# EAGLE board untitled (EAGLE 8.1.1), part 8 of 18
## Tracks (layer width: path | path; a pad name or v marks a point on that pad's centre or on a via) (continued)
S$7704 (continued)
  Bottom 0: 276.47,99.72 276.52,99.67
S$7705
  Bottom 0: 276.52,99.67 276.59,99.63
S$7706
  Bottom 0: 276.59,99.63 276.65,99.61
S$7707
  Bottom 0: 276.65,99.61 276.71,99.59
S$7708
  Bottom 0: 276.71,99.59 276.78,99.59
S$7709
  Bottom 0: 276.78,99.59 277.3,99.59
S$7710
  Bottom 0: 277.3,99.59 277.05,99.51
S$7711
  Bottom 0: 277.05,99.51 276.65,99.3
S$7712
  Bottom 0: 276.65,99.3 276.31,99.01
S$7713
  Bottom 0: 276.31,99.01 276.02,98.67
S$7714
  Bottom 0: 276.02,98.67 275.81,98.27
S$7715
  Bottom 0: 275.81,98.27 275.68,97.85
S$7716
  Bottom 0: 275.68,97.85 275.64,97.4
S$7717
  Bottom 0: 275.64,97.4 275.68,96.95
S$7718
  Bottom 0: 275.68,96.95 275.79,96.6
S$7719
  Bottom 0: 107.45,97.12 107.48,97.29
S$7720
  Bottom 0: 107.48,97.29 107.44,97.61
S$7721
  Bottom 0: 107.44,97.61 107.43,97.63
S$7722
  Bottom 0: 107.43,97.63 107.56,97.75
S$7723
  Bottom 0: 107.56,97.75 107.62,97.82
S$7724
  Bottom 0: 107.62,97.82 107.67,97.9
S$7725
  Bottom 0: 107.67,97.9 107.7,97.98
S$7726
  Bottom 0: 107.7,97.98 107.72,98.06
S$7727
  Bottom 0: 107.72,98.06 107.73,98.16
S$7728
  Bottom 0: 107.73,98.16 107.73,112.42
S$7729
  Bottom 0: 107.73,112.42 107.76,112.46
S$7730
  Bottom 0: 107.76,112.46 109.79,114.49
S$7731
  Bottom 0: 109.79,114.49 109.76,114.43
S$7732
  Bottom 0: 109.76,114.43 109.67,114.09
S$7733
  Bottom 0: 109.67,114.09 109.67,113.75
S$7734
  Bottom 0: 109.67,113.75 109.76,113.41
S$7735
  Bottom 0: 109.76,113.41 109.94,113.1
S$7736
  Bottom 0: 109.94,113.1 110.17,112.84
S$7737
  Bottom 0: 110.17,112.84 110.47,112.65
S$7738
  Bottom 0: 110.47,112.65 110.62,112.6
S$7739
  Bottom 0: 110.62,112.6 110.62,100.28
S$7740
  Bottom 0: 110.62,100.28 107.45,97.12
S$7741
  Bottom 0: 44.84,100.72 44.99,100.87
S$7742
  Bottom 0: 44.99,100.87 45.12,101.15
S$7743
  Bottom 0: 45.12,101.15 45.17,101.45
S$7744
  Bottom 0: 45.17,101.45 45.12,101.75
S$7745
  Bottom 0: 45.12,101.75 44.99,102.02
S$7746
  Bottom 0: 44.99,102.02 44.78,102.24
S$7747
  Bottom 0: 44.78,102.24 44.52,102.39
S$7748
  Bottom 0: 44.52,102.39 44.23,102.46
S$7749
  Bottom 0: 44.23,102.46 43.92,102.44
S$7750
  Bottom 0: 43.92,102.44 43.82,102.4
S$7751
  Bottom 0: 43.82,102.4 43.39,102.84
S$7752
  Bottom 0: 43.39,102.84 43.33,102.88
S$7753
  Bottom 0: 43.33,102.88 43.27,102.92
S$7754
  Bottom 0: 43.27,102.92 43.21,102.95
S$7755
  Bottom 0: 43.21,102.95 43.14,102.96
S$7756
  Bottom 0: 43.14,102.96 43.07,102.97
S$7757
  Bottom 0: 43.07,102.97 36.7,102.97
S$7758
  Bottom 0: 36.7,102.97 36.63,102.96
S$7759
  Bottom 0: 36.63,102.96 36.56,102.95
S$7760
  Bottom 0: 36.56,102.95 36.5,102.92
S$7761
  Bottom 0: 36.5,102.92 36.44,102.88
S$7762
  Bottom 0: 36.44,102.88 36.38,102.84
S$7763
  Bottom 0: 36.38,102.84 35.81,102.27
S$7764
  Bottom 0: 35.81,102.27 35.84,102.49
S$7765
  Bottom 0: 35.84,102.49 35.8,102.81
S$7766
  Bottom 0: 35.8,102.81 35.66,103.11
S$7767
  Bottom 0: 35.66,103.11 35.45,103.35
S$7768
  Bottom 0: 35.45,103.35 35.27,103.47
S$7769
  Bottom 0: 35.27,103.47 35.27,106.69
S$7770
  Bottom 0: 35.27,106.69 52.72,106.69
S$7771
  Bottom 0: 52.72,106.69 52.52,106.49
S$7772
  Bottom 0: 52.52,106.49 52.34,106.22
S$7773
  Bottom 0: 52.34,106.22 52.26,105.9
S$7774
  Bottom 0: 52.26,105.9 52.26,105.58
S$7775
  Bottom 0: 52.26,105.58 52.34,105.26
S$7776
  Bottom 0: 52.34,105.26 52.52,104.99
S$7777
  Bottom 0: 52.52,104.99 52.75,104.77
S$7778
  Bottom 0: 52.75,104.77 53.04,104.62
S$7779
  Bottom 0: 53.04,104.62 53.36,104.55
S$7780
  Bottom 0: 53.36,104.55 53.69,104.57
S$7781
  Bottom 0: 53.69,104.57 53.9,104.65
S$7782
  Bottom 0: 53.9,104.65 54.96,103.59
S$7783
  Bottom 0: 54.96,103.59 54.94,103.58
S$7784
  Bottom 0: 54.94,103.58 54.88,103.53
S$7785
  Bottom 0: 54.88,103.53 54.84,103.45
S$7786
  Bottom 0: 54.84,103.45 54.83,103.38
S$7787
  Bottom 0: 54.83,103.38 54.83,101.6
S$7788
  Bottom 0: 54.83,101.6 54.84,101.52
S$7789
  Bottom 0: 54.84,101.52 54.88,101.45
S$7790
  Bottom 0: 54.88,101.45 54.94,101.4
S$7791
  Bottom 0: 54.94,101.4 55.01,101.36
S$7792
  Bottom 0: 55.01,101.36 55.09,101.35
S$7793
  Bottom 0: 55.09,101.35 56.87,101.35
S$7794
  Bottom 0: 56.87,101.35 56.94,101.36
S$7795
  Bottom 0: 56.94,101.36 57.01,101.4
S$7796
  Bottom 0: 57.01,101.4 57.07,101.45
S$7797
  Bottom 0: 57.07,101.45 57.11,101.52
S$7798
  Bottom 0: 57.11,101.52 57.12,101.6
S$7799
  Bottom 0: 57.12,101.6 57.12,103.08
S$7800
  Bottom 0: 57.12,103.08 57.41,102.79
S$7801
  Bottom 0: 57.41,102.79 57.37,102.49
S$7802
  Bottom 0: 57.37,102.49 57.42,102.17
S$7803
  Bottom 0: 57.42,102.17 57.56,101.87
S$7804
  Bottom 0: 57.56,101.87 57.77,101.62
S$7805
  Bottom 0: 57.77,101.62 58.04,101.45
S$7806
  Bottom 0: 58.04,101.45 58.35,101.36
S$7807
  Bottom 0: 58.35,101.36 58.64,101.36
S$7808
  Bottom 0: 58.64,101.36 58,100.72
S$7809
  Bottom 0: 58,100.72 49.61,100.72
S$7810
  Bottom 0: 49.61,100.72 49.75,100.87
S$7811
  Bottom 0: 49.75,100.87 49.88,101.15
S$7812
  Bottom 0: 49.88,101.15 49.93,101.45
S$7813
  Bottom 0: 49.93,101.45 49.88,101.75
S$7814
  Bottom 0: 49.88,101.75 49.75,102.02
S$7815
  Bottom 0: 49.75,102.02 49.55,102.24
S$7816
  Bottom 0: 49.55,102.24 49.28,102.39
S$7817
  Bottom 0: 49.28,102.39 48.99,102.46
S$7818
  Bottom 0: 48.99,102.46 48.68,102.44
S$7819
  Bottom 0: 48.68,102.44 48.41,102.33
S$7820
  Bottom 0: 48.41,102.33 48.17,102.14
S$7821
  Bottom 0: 48.17,102.14 48,101.89
S$7822
  Bottom 0: 48,101.89 47.91,101.6
S$7823
  Bottom 0: 47.91,101.6 47.91,101.3
S$7824
  Bottom 0: 47.91,101.3 48,101.01
S$7825
  Bottom 0: 48,101.01 48.17,100.76
S$7826
  Bottom 0: 48.17,100.76 48.21,100.72
S$7827
  Bottom 0: 48.21,100.72 44.84,100.72
S$7828
  Bottom 0: 287.8,100.76 287.9,100.87
S$7829
  Bottom 0: 287.9,100.87 288.04,101.15
S$7830
  Bottom 0: 288.04,101.15 288.08,101.45
S$7831
  Bottom 0: 288.08,101.45 288.04,101.75
S$7832
  Bottom 0: 288.04,101.75 287.9,102.02
S$7833
  Bottom 0: 287.9,102.02 287.7,102.24
S$7834
  Bottom 0: 287.7,102.24 287.44,102.39
S$7835
  Bottom 0: 287.44,102.39 287.14,102.46
S$7836
  Bottom 0: 287.14,102.46 286.84,102.44
S$7837
  Bottom 0: 286.84,102.44 286.66,102.37
S$7838
  Bottom 0: 286.66,102.37 287.37,103.08
S$7839
  Bottom 0: 287.37,103.08 287.43,103.14
S$7840
  Bottom 0: 287.43,103.14 287.48,103.22
S$7841
  Bottom 0: 287.48,103.22 287.51,103.3
S$7842
  Bottom 0: 287.51,103.3 287.53,103.39
S$7843
  Bottom 0: 287.53,103.39 287.54,103.48
S$7844
  Bottom 0: 287.54,103.48 287.54,112.16
S$7845
  Bottom 0: 287.54,112.16 287.74,112
S$7846
  Bottom 0: 287.74,112 288.02,111.89
S$7847
  Bottom 0: 288.02,111.89 288.33,111.87
S$7848
  Bottom 0: 288.33,111.87 288.57,111.93
S$7849
  Bottom 0: 288.57,111.93 289.45,111.05
S$7850
  Bottom 0: 289.45,111.05 289.51,111
S$7851
  Bottom 0: 289.51,111 289.56,110.97
S$7852
  Bottom 0: 289.56,110.97 289.63,110.94
S$7853
  Bottom 0: 289.63,110.94 289.7,110.92
S$7854
  Bottom 0: 289.7,110.92 289.77,110.92
S$7855
  Bottom 0: 289.77,110.92 293.12,110.92
S$7856
  Bottom 0: 293.12,110.92 293.14,110.85
S$7857
  Bottom 0: 293.14,110.85 293.31,110.54
S$7858
  Bottom 0: 293.31,110.54 293.55,110.28
S$7859
  Bottom 0: 293.55,110.28 293.84,110.09
S$7860
  Bottom 0: 293.84,110.09 294.17,109.99
S$7861
  Bottom 0: 294.17,109.99 294.52,109.97
S$7862
  Bottom 0: 294.52,109.97 294.83,110.02
S$7863
  Bottom 0: 294.83,110.02 294.94,109.99
S$7864
  Bottom 0: 294.94,109.99 295.29,109.97
S$7865
  Bottom 0: 295.29,109.97 295.39,109.99
S$7866
  Bottom 0: 295.39,109.99 289.13,103.72
S$7867
  Bottom 0: 289.13,103.72 289.09,103.67
S$7868
  Bottom 0: 289.09,103.67 289.05,103.61
S$7869
  Bottom 0: 289.05,103.61 289.02,103.55
S$7870
  Bottom 0: 289.02,103.55 289.01,103.48
S$7871
  Bottom 0: 289.01,103.48 289,103.41
S$7872
  Bottom 0: 289,103.41 289,102.35
S$7873
  Bottom 0: 289,102.35 288.94,102.33
S$7874
  Bottom 0: 288.94,102.33 288.69,102.14
S$7875
  Bottom 0: 288.69,102.14 288.53,101.89
S$7876
  Bottom 0: 288.53,101.89 288.44,101.6
S$7877
  Bottom 0: 288.44,101.6 288.44,101.3
S$7878
  Bottom 0: 288.44,101.3 288.53,101.01
S$7879
  Bottom 0: 288.53,101.01 288.69,100.76
S$7880
  Bottom 0: 288.69,100.76 287.8,100.76
S$7881
  Bottom 0: 290.18,100.76 290.28,100.87
S$7882
  Bottom 0: 290.28,100.87 290.41,101.15
S$7883
  Bottom 0: 290.41,101.15 290.46,101.45
S$7884
  Bottom 0: 290.46,101.45 290.41,101.75
S$7885
  Bottom 0: 290.41,101.75 290.28,102.02
S$7886
  Bottom 0: 290.28,102.02 290.08,102.24
S$7887
  Bottom 0: 290.08,102.24 289.88,102.35
S$7888
  Bottom 0: 289.88,102.35 289.88,103.23
S$7889
  Bottom 0: 289.88,103.23 292.88,106.22
S$7890
  Bottom 0: 292.88,106.22 292.79,105.9
S$7891
  Bottom 0: 292.79,105.9 292.79,105.58
S$7892
  Bottom 0: 292.79,105.58 292.88,105.26
S$7893
  Bottom 0: 292.88,105.26 293.05,104.99
S$7894
  Bottom 0: 293.05,104.99 293.28,104.77
S$7895
  Bottom 0: 293.28,104.77 293.57,104.62
S$7896
  Bottom 0: 293.57,104.62 293.89,104.55
S$7897
  Bottom 0: 293.89,104.55 294.22,104.57
S$7898
  Bottom 0: 294.22,104.57 294.25,104.58
S$7899
  Bottom 0: 294.25,104.58 295.2,103.62
S$7900
  Bottom 0: 295.2,103.62 294.82,103.62
S$7901
  Bottom 0: 294.82,103.62 294.74,103.61
S$7902
  Bottom 0: 294.74,103.61 294.67,103.57
S$7903
  Bottom 0: 294.67,103.57 294.62,103.52
S$7904
  Bottom 0: 294.62,103.52 294.57,103.44
S$7905
  Bottom 0: 294.57,103.44 294.56,103.37
S$7906
  Bottom 0: 294.56,103.37 294.56,101.59
S$7907
  Bottom 0: 294.56,101.59 294.57,101.51
S$7908
  Bottom 0: 294.57,101.51 294.62,101.44
S$7909
  Bottom 0: 294.62,101.44 294.67,101.39
S$7910
  Bottom 0: 294.67,101.39 294.74,101.35
S$7911
  Bottom 0: 294.74,101.35 294.82,101.34
S$7912
  Bottom 0: 294.82,101.34 296.88,101.34
S$7913
  Bottom 0: 296.88,101.34 296.3,100.76
S$7914
  Bottom 0: 296.3,100.76 290.18,100.76
S$7915
  Bottom 0: 219.33,101.53 207.55,113.3
S$7916
  Bottom 0: 207.55,113.3 207.66,113.57
S$7917
  Bottom 0: 207.66,113.57 207.71,113.92
S$7918
  Bottom 0: 207.71,113.92 207.66,114.26
S$7919
  Bottom 0: 207.66,114.26 207.55,114.54
S$7920
  Bottom 0: 207.55,114.54 208.01,115
S$7921
  Bottom 0: 208.01,115 208.05,115.05
S$7922
  Bottom 0: 208.05,115.05 208.09,115.11
S$7923
  Bottom 0: 208.09,115.11 208.11,115.17
S$7924
  Bottom 0: 208.11,115.17 208.13,115.23
S$7925
  Bottom 0: 208.13,115.23 208.13,115.31
S$7926
  Bottom 0: 208.13,115.31 208.13,130.12
S$7927
  Bottom 0: 208.13,130.12 208.18,129.92
S$7928
  Bottom 0: 208.18,129.92 208.36,129.61
S$7929
  Bottom 0: 208.36,129.61 208.59,129.35
S$7930
  Bottom 0: 208.59,129.35 208.89,129.16
S$7931
  Bottom 0: 208.89,129.16 209.22,129.06
S$7932
  Bottom 0: 209.22,129.06 209.57,129.04
S$7933
  Bottom 0: 209.57,129.04 209.92,129.1
S$7934
  Bottom 0: 209.92,129.1 210.23,129.25
S$7935
  Bottom 0: 210.23,129.25 210.5,129.47
S$7936
  Bottom 0: 210.5,129.47 210.71,129.76
S$7937
  Bottom 0: 210.71,129.76 210.84,130.08
S$7938
  Bottom 0: 210.84,130.08 210.88,130.43
S$7939
  Bottom 0: 210.88,130.43 210.84,130.77
S$7940
  Bottom 0: 210.84,130.77 210.71,131.1
S$7941
  Bottom 0: 210.71,131.1 210.5,131.38
S$7942
  Bottom 0: 210.5,131.38 210.23,131.61
S$7943
  Bottom 0: 210.23,131.61 209.92,131.76
S$7944
  Bottom 0: 209.92,131.76 209.57,131.82
S$7945
  Bottom 0: 209.57,131.82 209.22,131.8
S$7946
  Bottom 0: 209.22,131.8 208.89,131.69
S$7947
  Bottom 0: 208.89,131.69 208.59,131.51
S$7948
  Bottom 0: 208.59,131.51 208.36,131.25
S$7949
  Bottom 0: 208.36,131.25 208.18,130.94
S$7950
  Bottom 0: 208.18,130.94 208.13,130.74
S$7951
  Bottom 0: 208.13,130.74 208.13,131.11
S$7952
  Bottom 0: 208.13,131.11 208.13,131.18
S$7953
  Bottom 0: 208.13,131.18 208.11,131.25
S$7954
  Bottom 0: 208.11,131.25 208.09,131.31
S$7955
  Bottom 0: 208.09,131.31 208.05,131.37
S$7956
  Bottom 0: 208.05,131.37 208.01,131.43
S$7957
  Bottom 0: 208.01,131.43 201.5,137.93
S$7958
  Bottom 0: 201.5,137.93 201.51,137.98
S$7959
  Bottom 0: 201.51,137.98 201.47,138.23
S$7960
  Bottom 0: 201.47,138.23 201.34,138.44
S$7961
  Bottom 0: 201.34,138.44 201.13,138.59
S$7962
  Bottom 0: 201.13,138.59 200.89,138.66
S$7963
  Bottom 0: 200.89,138.66 200.64,138.64
S$7964
  Bottom 0: 200.64,138.64 200.42,138.53
S$7965
  Bottom 0: 200.42,138.53 200.24,138.34
S$7966
  Bottom 0: 200.24,138.34 200.15,138.1
S$7967
  Bottom 0: 200.15,138.1 200.15,138.03
S$7968
  Bottom 0: 200.15,138.03 195.97,142.21
S$7969
  Bottom 0: 195.97,142.21 196.47,142.7
S$7970
  Bottom 0: 196.47,142.7 196.72,142.65
S$7971
  Bottom 0: 196.72,142.65 197.05,142.67
S$7972
  Bottom 0: 197.05,142.67 197.35,142.78
S$7973
  Bottom 0: 197.35,142.78 197.62,142.97
S$7974
  Bottom 0: 197.62,142.97 197.82,143.22
S$7975
  Bottom 0: 197.82,143.22 197.95,143.52
S$7976
  Bottom 0: 197.95,143.52 198,143.84
S$7977
  Bottom 0: 198,143.84 197.95,144.16
S$7978
  Bottom 0: 197.95,144.16 197.82,144.46
S$7979
  Bottom 0: 197.82,144.46 197.62,144.71
S$7980
  Bottom 0: 197.62,144.71 197.35,144.9
S$7981
  Bottom 0: 197.35,144.9 197.05,145.01
S$7982
  Bottom 0: 197.05,145.01 196.72,145.03
S$7983
  Bottom 0: 196.72,145.03 196.4,144.96
S$7984
  Bottom 0: 196.4,144.96 196.11,144.82
S$7985
  Bottom 0: 196.11,144.82 195.88,144.59
S$7986
  Bottom 0: 195.88,144.59 195.71,144.32
S$7987
  Bottom 0: 195.71,144.32 195.62,144
S$7988
  Bottom 0: 195.62,144 195.62,143.68
S$7989
  Bottom 0: 195.62,143.68 195.66,143.51
S$7990
  Bottom 0: 195.66,143.51 194.94,142.78
S$7991
  Bottom 0: 194.94,142.78 189.73,142.78
S$7992
  Bottom 0: 189.73,142.78 190,142.97
S$7993
  Bottom 0: 190,142.97 190.2,143.22
S$7994
  Bottom 0: 190.2,143.22 190.33,143.52
S$7995
  Bottom 0: 190.33,143.52 190.38,143.84
S$7996
  Bottom 0: 190.38,143.84 190.33,144.16
S$7997
  Bottom 0: 190.33,144.16 190.2,144.46
S$7998
  Bottom 0: 190.2,144.46 190,144.71
S$7999
  Bottom 0: 190,144.71 189.73,144.9
S$8000
  Bottom 0: 189.73,144.9 189.43,145.01
S$8001
  Bottom 0: 189.43,145.01 189.1,145.03
S$8002
  Bottom 0: 189.1,145.03 188.78,144.96
S$8003
  Bottom 0: 188.78,144.96 188.49,144.82
S$8004
  Bottom 0: 188.49,144.82 188.26,144.59
S$8005
  Bottom 0: 188.26,144.59 188.09,144.32
S$8006
  Bottom 0: 188.09,144.32 188,144
S$8007
  Bottom 0: 188,144 188,143.68
S$8008
  Bottom 0: 188,143.68 188.09,143.36
S$8009
  Bottom 0: 188.09,143.36 188.26,143.09
S$8010
  Bottom 0: 188.26,143.09 188.49,142.87
S$8011
  Bottom 0: 188.49,142.87 188.66,142.78
S$8012
  Bottom 0: 188.66,142.78 179.62,142.78
S$8013
  Bottom 0: 179.62,142.78 178.9,143.5
S$8014
  Bottom 0: 178.9,143.5 178.9,143.52
S$8015
  Bottom 0: 178.9,143.52 178.95,143.84
S$8016
  Bottom 0: 178.95,143.84 178.9,144.16
S$8017
  Bottom 0: 178.9,144.16 178.77,144.46
S$8018
  Bottom 0: 178.77,144.46 178.57,144.71
S$8019
  Bottom 0: 178.57,144.71 178.3,144.9
S$8020
  Bottom 0: 178.3,144.9 178,145.01
S$8021
  Bottom 0: 178,145.01 177.67,145.03
S$8022
  Bottom 0: 177.67,145.03 177.35,144.96
S$8023
  Bottom 0: 177.35,144.96 177.06,144.82
S$8024
  Bottom 0: 177.06,144.82 176.83,144.59
S$8025
  Bottom 0: 176.83,144.59 176.66,144.32
S$8026
  Bottom 0: 176.66,144.32 176.57,144
S$8027
  Bottom 0: 176.57,144 176.57,143.68
S$8028
  Bottom 0: 176.57,143.68 176.66,143.36
S$8029
  Bottom 0: 176.66,143.36 176.83,143.09
S$8030
  Bottom 0: 176.83,143.09 177.06,142.87
S$8031
  Bottom 0: 177.06,142.87 177.35,142.72
S$8032
  Bottom 0: 177.35,142.72 177.67,142.65
S$8033
  Bottom 0: 177.67,142.65 178,142.67
S$8034
  Bottom 0: 178,142.67 178.09,142.7
S$8035
  Bottom 0: 178.09,142.7 178.82,141.98
S$8036
  Bottom 0: 178.82,141.98 178.82,133.83
S$8037
  Bottom 0: 178.82,133.83 178.75,133.92
S$8038
  Bottom 0: 178.75,133.92 178.48,134.15
S$8039
  Bottom 0: 178.48,134.15 178.18,134.29
S$8040
  Bottom 0: 178.18,134.29 178.18,140.53
S$8041
  Bottom 0: 178.18,140.53 178.17,140.6
S$8042
  Bottom 0: 178.17,140.6 178.16,140.66
S$8043
  Bottom 0: 178.16,140.66 178.13,140.73
S$8044
  Bottom 0: 178.13,140.73 178.09,140.79
S$8045
  Bottom 0: 178.09,140.79 178.05,140.84
S$8046
  Bottom 0: 178.05,140.84 173.08,145.81
S$8047
  Bottom 0: 173.08,145.81 173.09,145.86
S$8048
  Bottom 0: 173.09,145.86 173.04,146.11
S$8049
  Bottom 0: 173.04,146.11 172.91,146.32
S$8050
  Bottom 0: 172.91,146.32 172.71,146.48
S$8051
  Bottom 0: 172.71,146.48 172.46,146.54
S$8052
  Bottom 0: 172.46,146.54 172.21,146.52
S$8053
  Bottom 0: 172.21,146.52 171.99,146.41
S$8054
  Bottom 0: 171.99,146.41 171.82,146.22
S$8055
  Bottom 0: 171.82,146.22 171.72,145.99
S$8056
  Bottom 0: 171.72,145.99 171.72,145.74
S$8057
  Bottom 0: 171.72,145.74 171.82,145.5
S$8058
  Bottom 0: 171.82,145.5 171.99,145.31
S$8059
  Bottom 0: 171.99,145.31 172.21,145.2
S$8060
  Bottom 0: 172.21,145.2 172.45,145.18
S$8061
  Bottom 0: 172.45,145.18 177.29,140.34
S$8062
  Bottom 0: 177.29,140.34 177.29,134.28
S$8063
  Bottom 0: 177.29,134.28 177.14,134.23
S$8064
  Bottom 0: 177.14,134.23 176.84,134.05
S$8065
  Bottom 0: 176.84,134.05 176.61,133.79
S$8066
  Bottom 0: 176.61,133.79 176.43,133.48
S$8067
  Bottom 0: 176.43,133.48 176.35,133.14
S$8068
  Bottom 0: 176.35,133.14 176.35,132.79
S$8069
  Bottom 0: 176.35,132.79 176.43,132.46
S$8070
  Bottom 0: 176.43,132.46 176.61,132.15
S$8071
  Bottom 0: 176.61,132.15 176.84,131.89
S$8072
  Bottom 0: 176.84,131.89 177.14,131.7
S$8073
  Bottom 0: 177.14,131.7 177.47,131.6
S$8074
  Bottom 0: 177.47,131.6 177.82,131.58
S$8075
  Bottom 0: 177.82,131.58 178.17,131.64
S$8076
  Bottom 0: 178.17,131.64 178.48,131.79
S$8077
  Bottom 0: 178.48,131.79 178.75,132.01
S$8078
  Bottom 0: 178.75,132.01 178.82,132.11
S$8079
  Bottom 0: 178.82,132.11 178.82,127.99
S$8080
  Bottom 0: 178.82,127.99 177.69,126.86
S$8081
  Bottom 0: 177.69,126.86 177.63,126.79
S$8082
  Bottom 0: 177.63,126.79 177.58,126.72
S$8083
  Bottom 0: 177.58,126.72 177.55,126.63
S$8084
  Bottom 0: 177.55,126.63 177.53,126.55
S$8085
  Bottom 0: 177.53,126.55 177.52,126.46
S$8086
  Bottom 0: 177.52,126.46 177.52,123.5
S$8087
  Bottom 0: 177.52,123.5 170.33,123.5
S$8088
  Bottom 0: 170.33,123.5 169.37,124.45
S$8089
  Bottom 0: 169.37,124.45 169.38,124.47
S$8090
  Bottom 0: 169.38,124.47 169.42,124.79
S$8091
  Bottom 0: 169.42,124.79 169.38,125.11
S$8092
  Bottom 0: 169.38,125.11 169.25,125.41
S$8093
  Bottom 0: 169.25,125.41 169.04,125.66
S$8094
  Bottom 0: 169.04,125.66 168.78,125.85
S$8095
  Bottom 0: 168.78,125.85 168.47,125.96
S$8096
  Bottom 0: 168.47,125.96 168.15,125.98
S$8097
  Bottom 0: 168.15,125.98 167.83,125.91
S$8098
  Bottom 0: 167.83,125.91 167.69,125.84
S$8099
  Bottom 0: 167.69,125.84 161.02,132.52
S$8100
  Bottom 0: 161.02,132.52 161.02,142.1
S$8101
  Bottom 0: 161.02,142.1 161.01,142.19
S$8102
  Bottom 0: 161.01,142.19 161,142.28
S$8103
  Bottom 0: 161,142.28 160.96,142.36
S$8104
  Bottom 0: 160.96,142.36 160.91,142.43
S$8105
  Bottom 0: 160.91,142.43 160.85,142.5
S$8106
  Bottom 0: 160.85,142.5 159.85,143.5
S$8107
  Bottom 0: 159.85,143.5 159.85,143.52
S$8108
  Bottom 0: 159.85,143.52 159.9,143.84
S$8109
  Bottom 0: 159.9,143.84 159.85,144.16
S$8110
  Bottom 0: 159.85,144.16 159.72,144.47
S$8111
  Bottom 0: 159.72,144.47 159.52,144.72
S$8112
  Bottom 0: 159.52,144.72 159.25,144.91
S$8113
  Bottom 0: 159.25,144.91 158.95,145.01
S$8114
  Bottom 0: 158.95,145.01 158.62,145.03
S$8115
  Bottom 0: 158.62,145.03 158.3,144.97
S$8116
  Bottom 0: 158.3,144.97 158.01,144.82
S$8117
  Bottom 0: 158.01,144.82 157.78,144.6
S$8118
  Bottom 0: 157.78,144.6 157.61,144.32
S$8119
  Bottom 0: 157.61,144.32 157.52,144.01
S$8120
  Bottom 0: 157.52,144.01 157.52,143.68
S$8121
  Bottom 0: 157.52,143.68 157.61,143.37
S$8122
  Bottom 0: 157.61,143.37 157.78,143.09
S$8123
  Bottom 0: 157.78,143.09 158.01,142.87
S$8124
  Bottom 0: 158.01,142.87 158.3,142.72
S$8125
  Bottom 0: 158.3,142.72 158.62,142.66
S$8126
  Bottom 0: 158.62,142.66 158.95,142.68
S$8127
  Bottom 0: 158.95,142.68 159.04,142.71
S$8128
  Bottom 0: 159.04,142.71 159.88,141.86
S$8129
  Bottom 0: 159.88,141.86 159.88,133.68
S$8130
  Bottom 0: 159.88,133.68 159.7,133.92
S$8131
  Bottom 0: 159.7,133.92 159.43,134.15
S$8132
  Bottom 0: 159.43,134.15 159.13,134.29
S$8133
  Bottom 0: 159.13,134.29 159.13,141.39
S$8134
  Bottom 0: 159.13,141.39 159.12,141.46
S$8135
  Bottom 0: 159.12,141.46 159.11,141.53
S$8136
  Bottom 0: 159.11,141.53 159.08,141.59
S$8137
  Bottom 0: 159.08,141.59 159.04,141.65
S$8138
  Bottom 0: 159.04,141.65 158.99,141.71
S$8139
  Bottom 0: 158.99,141.71 155.73,144.97
S$8140
  Bottom 0: 155.73,144.97 155.74,145.02
S$8141
  Bottom 0: 155.74,145.02 155.69,145.27
S$8142
  Bottom 0: 155.69,145.27 155.56,145.48
S$8143
  Bottom 0: 155.56,145.48 155.36,145.63
S$8144
  Bottom 0: 155.36,145.63 155.11,145.7
S$8145
  Bottom 0: 155.11,145.7 154.86,145.68
S$8146
  Bottom 0: 154.86,145.68 154.64,145.57
S$8147
  Bottom 0: 154.64,145.57 154.6,145.53
S$8148
  Bottom 0: 154.6,145.53 154.6,145.89
S$8149
  Bottom 0: 154.6,145.89 156.11,147.39
S$8150
  Bottom 0: 156.11,147.39 168.79,147.39
S$8151
  Bottom 0: 168.79,147.39 168.86,147.4
S$8152
  Bottom 0: 168.86,147.4 168.93,147.42
S$8153
  Bottom 0: 168.93,147.42 168.99,147.44
S$8154
  Bottom 0: 168.99,147.44 169.05,147.48
S$8155
  Bottom 0: 169.05,147.48 169.11,147.52
S$8156
  Bottom 0: 169.11,147.52 172.35,150.77
S$8157
  Bottom 0: 172.35,150.77 172.38,150.75
S$8158
  Bottom 0: 172.38,150.75 172.71,150.65
S$8159
  Bottom 0: 172.71,150.65 173.06,150.63
S$8160
  Bottom 0: 173.06,150.63 173.41,150.69
S$8161
  Bottom 0: 173.41,150.69 173.59,150.78
S$8162
  Bottom 0: 173.59,150.78 177.79,146.57
S$8163
  Bottom 0: 177.79,146.57 177.85,146.53
S$8164
  Bottom 0: 177.85,146.53 177.9,146.49
S$8165
  Bottom 0: 177.9,146.49 177.97,146.46
S$8166
  Bottom 0: 177.97,146.46 178.03,146.44
S$8167
  Bottom 0: 178.03,146.44 178.1,146.44
S$8168
  Bottom 0: 178.1,146.44 196.85,146.44
S$8169
  Bottom 0: 196.85,146.44 202.78,140.52
S$8170
  Bottom 0: 202.78,140.52 202.59,140.56
S$8171
  Bottom 0: 202.59,140.56 202.29,140.54
S$8172
  Bottom 0: 202.29,140.54 202.01,140.43
S$8173
  Bottom 0: 202.01,140.43 201.77,140.24
S$8174
  Bottom 0: 201.77,140.24 201.6,140
S$8175
  Bottom 0: 201.6,140 201.51,139.71
S$8176
  Bottom 0: 201.51,139.71 201.51,139.4
S$8177
  Bottom 0: 201.51,139.4 201.6,139.11
S$8178
  Bottom 0: 201.6,139.11 201.77,138.86
S$8179
  Bottom 0: 201.77,138.86 202.01,138.67
S$8180
  Bottom 0: 202.01,138.67 202.29,138.56
S$8181
  Bottom 0: 202.29,138.56 202.59,138.54
S$8182
  Bottom 0: 202.59,138.54 202.89,138.61
S$8183
  Bottom 0: 202.89,138.61 203.15,138.76
S$8184
  Bottom 0: 203.15,138.76 203.35,138.98
S$8185
  Bottom 0: 203.35,138.98 203.49,139.25
S$8186
  Bottom 0: 203.49,139.25 203.53,139.55
S$8187
  Bottom 0: 203.53,139.55 203.5,139.8
S$8188
  Bottom 0: 203.5,139.8 205.7,137.6
S$8189
  Bottom 0: 205.7,137.6 205.76,137.55
S$8190
  Bottom 0: 205.76,137.55 205.82,137.52
S$8191
  Bottom 0: 205.82,137.52 205.88,137.49
S$8192
  Bottom 0: 205.88,137.49 205.95,137.47
S$8193
  Bottom 0: 205.95,137.47 206.02,137.47
S$8194
  Bottom 0: 206.02,137.47 210.87,137.47
S$8195
  Bottom 0: 210.87,137.47 210.75,137.41
S$8196
  Bottom 0: 210.75,137.41 210.41,137.12
S$8197
  Bottom 0: 210.41,137.12 210.12,136.78
S$8198
  Bottom 0: 210.12,136.78 209.91,136.38
S$8199
  Bottom 0: 209.91,136.38 209.78,135.96
S$8200
  Bottom 0: 209.78,135.96 209.74,135.51
S$8201
  Bottom 0: 209.74,135.51 209.78,135.06
S$8202
  Bottom 0: 209.78,135.06 209.91,134.63
S$8203
  Bottom 0: 209.91,134.63 210.12,134.24
S$8204
  Bottom 0: 210.12,134.24 210.41,133.89
S$8205
  Bottom 0: 210.41,133.89 210.75,133.61
S$8206
  Bottom 0: 210.75,133.61 211.15,133.4
S$8207
  Bottom 0: 211.15,133.4 211.58,133.27
S$8208
  Bottom 0: 211.58,133.27 212.02,133.22
S$8209
  Bottom 0: 212.02,133.22 212.47,133.27
S$8210
  Bottom 0: 212.47,133.27 212.9,133.4
S$8211
  Bottom 0: 212.9,133.4 213.29,133.61
S$8212
  Bottom 0: 213.29,133.61 213.64,133.89
S$8213
  Bottom 0: 213.64,133.89 213.92,134.24
S$8214
  Bottom 0: 213.92,134.24 214.14,134.63
S$8215
  Bottom 0: 214.14,134.63 214.26,135.06
S$8216
  Bottom 0: 214.26,135.06 214.31,135.51
S$8217
  Bottom 0: 214.31,135.51 214.26,135.96
S$8218
  Bottom 0: 214.26,135.96 214.23,136.07
S$8219
  Bottom 0: 214.23,136.07 215.39,134.91
S$8220
  Bottom 0: 215.39,134.91 215.39,134.28
S$8221
  Bottom 0: 215.39,134.28 215.24,134.23
S$8222
  Bottom 0: 215.24,134.23 214.94,134.05
S$8223
  Bottom 0: 214.94,134.05 214.71,133.79
S$8224
  Bottom 0: 214.71,133.79 214.53,133.48
S$8225
  Bottom 0: 214.53,133.48 214.45,133.14
S$8226
  Bottom 0: 214.45,133.14 214.45,132.79
S$8227
  Bottom 0: 214.45,132.79 214.53,132.46
S$8228
  Bottom 0: 214.53,132.46 214.71,132.15
S$8229
  Bottom 0: 214.71,132.15 214.94,131.89
S$8230
  Bottom 0: 214.94,131.89 215.24,131.7
S$8231
  Bottom 0: 215.24,131.7 215.57,131.6
S$8232
  Bottom 0: 215.57,131.6 215.92,131.58
S$8233
  Bottom 0: 215.92,131.58 216.27,131.64
S$8234
  Bottom 0: 216.27,131.64 216.58,131.79
S$8235
  Bottom 0: 216.58,131.79 216.85,132.01
S$8236
  Bottom 0: 216.85,132.01 217.06,132.3
S$8237
  Bottom 0: 217.06,132.3 217.19,132.62
S$8238
  Bottom 0: 217.19,132.62 217.23,132.97
S$8239
  Bottom 0: 217.23,132.97 217.19,133.31
S$8240
  Bottom 0: 217.19,133.31 217.17,133.35
S$8241
  Bottom 0: 217.17,133.35 222.1,128.42
S$8242
  Bottom 0: 222.1,128.42 222.1,122.42
S$8243
  Bottom 0: 222.1,122.42 222.07,122.4
S$8244
  Bottom 0: 222.07,122.4 221.86,122.16
S$8245
  Bottom 0: 221.86,122.16 221.72,121.86
S$8246
  Bottom 0: 221.72,121.86 221.68,121.54
S$8247
  Bottom 0: 221.68,121.54 221.72,121.24
S$8248
  Bottom 0: 221.72,121.24 221.42,120.95
S$8249
  Bottom 0: 221.42,120.95 221.42,122.43
S$8250
  Bottom 0: 221.42,122.43 221.41,122.5
S$8251
  Bottom 0: 221.41,122.5 221.37,122.58
S$8252
  Bottom 0: 221.37,122.58 221.31,122.63
S$8253
  Bottom 0: 221.31,122.63 221.24,122.67
S$8254
  Bottom 0: 221.24,122.67 221.17,122.68
S$8255
  Bottom 0: 221.17,122.68 220.72,122.68
S$8256
  Bottom 0: 220.72,122.68 220.72,122.81
S$8257
  Bottom 0: 220.72,122.81 220.66,123.03
S$8258
  Bottom 0: 220.66,123.03 220.5,123.19
S$8259
  Bottom 0: 220.5,123.19 220.28,123.25
S$8260
  Bottom 0: 220.28,123.25 219.93,123.25
S$8261
  Bottom 0: 219.93,123.25 218.85,124.33
S$8262
  Bottom 0: 218.85,124.33 218.91,124.47
S$8263
  Bottom 0: 218.91,124.47 218.96,124.79
S$8264
  Bottom 0: 218.96,124.79 218.91,125.11
S$8265
  Bottom 0: 218.91,125.11 218.78,125.41
S$8266
  Bottom 0: 218.78,125.41 218.58,125.66
S$8267
  Bottom 0: 218.58,125.66 218.31,125.85
S$8268
  Bottom 0: 218.31,125.85 218.01,125.96
S$8269
  Bottom 0: 218.01,125.96 217.68,125.98
S$8270
  Bottom 0: 217.68,125.98 217.36,125.91
S$8271
  Bottom 0: 217.36,125.91 217.07,125.77
S$8272
  Bottom 0: 217.07,125.77 216.84,125.54
S$8273
  Bottom 0: 216.84,125.54 216.67,125.27
S$8274
  Bottom 0: 216.67,125.27 216.58,124.95
S$8275
  Bottom 0: 216.58,124.95 216.58,124.63
S$8276
  Bottom 0: 216.58,124.63 216.67,124.31
S$8277
  Bottom 0: 216.67,124.31 216.84,124.04
S$8278
  Bottom 0: 216.84,124.04 217.07,123.81
S$8279
  Bottom 0: 217.07,123.81 217.36,123.67
S$8280
  Bottom 0: 217.36,123.67 217.68,123.6
S$8281
  Bottom 0: 217.68,123.6 218.01,123.62
S$8282
  Bottom 0: 218.01,123.62 218.23,123.7
S$8283
  Bottom 0: 218.23,123.7 219.27,122.65
S$8284
  Bottom 0: 219.27,122.65 219.24,122.63
S$8285
  Bottom 0: 219.24,122.63 219.19,122.58
S$8286
  Bottom 0: 219.19,122.58 219.15,122.5
S$8287
  Bottom 0: 219.15,122.5 219.14,122.43
S$8288
  Bottom 0: 219.14,122.43 219.14,120.65
S$8289
  Bottom 0: 219.14,120.65 219.15,120.57
S$8290
  Bottom 0: 219.15,120.57 219.19,120.5
S$8291
  Bottom 0: 219.19,120.5 219.24,120.45
S$8292
  Bottom 0: 219.24,120.45 219.31,120.41
S$8293
  Bottom 0: 219.31,120.41 219.39,120.4
S$8294
  Bottom 0: 219.39,120.4 220.87,120.4
S$8295
  Bottom 0: 220.87,120.4 216.94,116.46
S$8296
  Bottom 0: 216.94,116.46 216.88,116.4
S$8297
  Bottom 0: 216.88,116.4 216.84,116.32
S$8298
  Bottom 0: 216.84,116.32 216.8,116.24
S$8299
  Bottom 0: 216.8,116.24 216.78,116.15
S$8300
  Bottom 0: 216.78,116.15 216.77,116.06
S$8301
  Bottom 0: 216.77,116.06 216.77,110.4
S$8302
  Bottom 0: 216.77,110.4 216.78,110.32
S$8303
  Bottom 0: 216.78,110.32 216.8,110.23
S$8304
  Bottom 0: 216.8,110.23 216.84,110.14
S$8305
  Bottom 0: 216.84,110.14 216.88,110.07
S$8306
  Bottom 0: 216.88,110.07 216.94,110
S$8307
  Bottom 0: 216.94,110 217.95,108.99
S$8308
  Bottom 0: 217.95,108.99 218.02,108.93
S$8309
  Bottom 0: 218.02,108.93 218.09,108.88
S$8310
  Bottom 0: 218.09,108.88 218.18,108.85
S$8311
  Bottom 0: 218.18,108.85 218.26,108.82
S$8312
  Bottom 0: 218.26,108.82 218.35,108.82
S$8313
  Bottom 0: 218.35,108.82 218.45,108.82
S$8314
  Bottom 0: 218.45,108.82 220.36,106.91
S$8315
  Bottom 0: 220.36,106.91 220.07,106.93
S$8316
  Bottom 0: 220.07,106.93 219.75,106.86
S$8317
  Bottom 0: 219.75,106.86 219.46,106.72
S$8318
  Bottom 0: 219.46,106.72 219.22,106.49
S$8319
  Bottom 0: 219.22,106.49 219.05,106.22
S$8320
  Bottom 0: 219.05,106.22 218.96,105.9
S$8321
  Bottom 0: 218.96,105.9 218.96,105.58
S$8322
  Bottom 0: 218.96,105.58 219.05,105.26
S$8323
  Bottom 0: 219.05,105.26 219.22,104.99
S$8324
  Bottom 0: 219.22,104.99 219.46,104.77
S$8325
  Bottom 0: 219.46,104.77 219.75,104.62
S$8326
  Bottom 0: 219.75,104.62 220.07,104.55
S$8327
  Bottom 0: 220.07,104.55 220.39,104.57
S$8328
  Bottom 0: 220.39,104.57 220.61,104.65
S$8329
  Bottom 0: 220.61,104.65 221.66,103.6
S$8330
  Bottom 0: 221.66,103.6 221.62,103.58
S$8331
  Bottom 0: 221.62,103.58 221.57,103.53
S$8332
  Bottom 0: 221.57,103.53 221.53,103.45
S$8333
  Bottom 0: 221.53,103.45 221.52,103.38
S$8334
  Bottom 0: 221.52,103.38 221.52,101.6
S$8335
  Bottom 0: 221.52,101.6 221.53,101.53
S$8336
  Bottom 0: 221.53,101.53 219.33,101.53
S$8337
  Bottom 0: 212.12,111.87 212.41,111.94
S$8338
  Bottom 0: 212.41,111.94 212.68,112.09
S$8339
  Bottom 0: 212.68,112.09 212.88,112.31
S$8340
  Bottom 0: 212.88,112.31 213.01,112.58
S$8341
  Bottom 0: 213.01,112.58 213.06,112.88
S$8342
  Bottom 0: 213.06,112.88 213.01,113.18
S$8343
  Bottom 0: 213.01,113.18 212.88,113.46
S$8344
  Bottom 0: 212.88,113.46 212.68,113.67
S$8345
  Bottom 0: 212.68,113.67 212.41,113.83
S$8346
  Bottom 0: 212.41,113.83 212.12,113.89
S$8347
  Bottom 0: 212.12,113.89 211.82,113.87
S$8348
  Bottom 0: 211.82,113.87 211.54,113.76
S$8349
  Bottom 0: 211.54,113.76 211.3,113.57
S$8350
  Bottom 0: 211.3,113.57 211.13,113.33
S$8351
  Bottom 0: 211.13,113.33 211.04,113.03
S$8352
  Bottom 0: 211.04,113.03 211.04,112.73
S$8353
  Bottom 0: 211.04,112.73 211.13,112.44
S$8354
  Bottom 0: 211.13,112.44 211.3,112.19
S$8355
  Bottom 0: 211.3,112.19 211.54,112
S$8356
  Bottom 0: 211.54,112 211.82,111.89
S$8357
  Bottom 0: 211.82,111.89 212.12,111.87
S$8358
  Bottom 0: 212.12,119.49 212.41,119.56
S$8359
  Bottom 0: 212.41,119.56 212.68,119.71
S$8360
  Bottom 0: 212.68,119.71 212.88,119.93
S$8361
  Bottom 0: 212.88,119.93 213.01,120.2
S$8362
  Bottom 0: 213.01,120.2 213.06,120.5
S$8363
  Bottom 0: 213.06,120.5 213.01,120.8
S$8364
  Bottom 0: 213.01,120.8 212.88,121.08
S$8365
  Bottom 0: 212.88,121.08 212.68,121.3
S$8366
  Bottom 0: 212.68,121.3 212.41,121.45
S$8367
  Bottom 0: 212.41,121.45 212.12,121.51
S$8368
  Bottom 0: 212.12,121.51 211.82,121.49
S$8369
  Bottom 0: 211.82,121.49 211.54,121.38
S$8370
  Bottom 0: 211.54,121.38 211.3,121.19
S$8371
  Bottom 0: 211.3,121.19 211.13,120.94
S$8372
  Bottom 0: 211.13,120.94 211.04,120.66
S$8373
  Bottom 0: 211.04,120.66 211.04,120.35
S$8374
  Bottom 0: 211.04,120.35 211.13,120.06
S$8375
  Bottom 0: 211.13,120.06 211.3,119.81
S$8376
  Bottom 0: 211.3,119.81 211.54,119.62
S$8377
  Bottom 0: 211.54,119.62 211.82,119.51
S$8378
  Bottom 0: 211.82,119.51 212.12,119.49
S$8379
  Bottom 0: 171.47,129.04 171.82,129.1
S$8380
  Bottom 0: 171.82,129.1 172.13,129.25
S$8381
  Bottom 0: 172.13,129.25 172.4,129.47
S$8382
  Bottom 0: 172.4,129.47 172.61,129.76
S$8383
  Bottom 0: 172.61,129.76 172.74,130.08
S$8384
  Bottom 0: 172.74,130.08 172.78,130.43
S$8385
  Bottom 0: 172.78,130.43 172.74,130.77
S$8386
  Bottom 0: 172.74,130.77 172.61,131.1
S$8387
  Bottom 0: 172.61,131.1 172.4,131.38
S$8388
  Bottom 0: 172.4,131.38 172.13,131.61
S$8389
  Bottom 0: 172.13,131.61 171.82,131.76
S$8390
  Bottom 0: 171.82,131.76 171.47,131.82
S$8391
  Bottom 0: 171.47,131.82 171.12,131.8
S$8392
  Bottom 0: 171.12,131.8 170.79,131.69
S$8393
  Bottom 0: 170.79,131.69 170.76,131.68
S$8394
  Bottom 0: 170.76,131.68 170.19,132.25
S$8395
  Bottom 0: 170.19,132.25 170.14,132.29
S$8396
  Bottom 0: 170.14,132.29 170.08,132.33
S$8397
  Bottom 0: 170.08,132.33 170.01,132.35
S$8398
  Bottom 0: 170.01,132.35 169.95,132.37
S$8399
  Bottom 0: 169.95,132.37 169.88,132.38
S$8400
  Bottom 0: 169.88,132.38 165.32,132.38
S$8401
  Bottom 0: 165.32,132.38 165.26,132.51
S$8402
  Bottom 0: 165.26,132.51 165.05,132.72
S$8403
  Bottom 0: 165.05,132.72 164.79,132.88
S$8404
  Bottom 0: 164.79,132.88 164.5,132.94
S$8405
  Bottom 0: 164.5,132.94 164.19,132.92
S$8406
  Bottom 0: 164.19,132.92 163.91,132.81
S$8407
  Bottom 0: 163.91,132.81 163.67,132.62
S$8408
  Bottom 0: 163.67,132.62 163.5,132.38
S$8409
  Bottom 0: 163.5,132.38 163.41,132.09
S$8410
  Bottom 0: 163.41,132.09 163.41,131.78
S$8411
  Bottom 0: 163.41,131.78 163.5,131.49
S$8412
  Bottom 0: 163.5,131.49 163.67,131.24
S$8413
  Bottom 0: 163.67,131.24 163.91,131.05
S$8414
  Bottom 0: 163.91,131.05 164.19,130.94
S$8415
  Bottom 0: 164.19,130.94 164.5,130.92
S$8416
  Bottom 0: 164.5,130.92 164.79,130.99
S$8417
  Bottom 0: 164.79,130.99 165.05,131.14
S$8418
  Bottom 0: 165.05,131.14 165.26,131.36
S$8419
  Bottom 0: 165.26,131.36 165.32,131.49
S$8420
  Bottom 0: 165.32,131.49 169.69,131.49
S$8421
  Bottom 0: 169.69,131.49 170.14,131.04
S$8422
  Bottom 0: 170.14,131.04 170.08,130.94
S$8423
  Bottom 0: 170.08,130.94 170,130.6
S$8424
  Bottom 0: 170,130.6 170,130.25
S$8425
  Bottom 0: 170,130.25 170.08,129.92
S$8426
  Bottom 0: 170.08,129.92 170.26,129.61
S$8427
  Bottom 0: 170.26,129.61 170.5,129.35
S$8428
  Bottom 0: 170.5,129.35 170.79,129.16
S$8429
  Bottom 0: 170.79,129.16 171.12,129.06
S$8430
  Bottom 0: 171.12,129.06 171.47,129.04
S$8431
  Bottom 0: 173.92,133.22 174.37,133.27
S$8432
  Bottom 0: 174.37,133.27 174.8,133.4
S$8433
  Bottom 0: 174.8,133.4 175.19,133.61
S$8434
  Bottom 0: 175.19,133.61 175.54,133.89
S$8435
  Bottom 0: 175.54,133.89 175.82,134.24
S$8436
  Bottom 0: 175.82,134.24 176.04,134.63
S$8437
  Bottom 0: 176.04,134.63 176.16,135.06
S$8438
  Bottom 0: 176.16,135.06 176.21,135.51
S$8439
  Bottom 0: 176.21,135.51 176.16,135.96
S$8440
  Bottom 0: 176.16,135.96 176.04,136.38
S$8441
  Bottom 0: 176.04,136.38 175.82,136.78
S$8442
  Bottom 0: 175.82,136.78 175.54,137.12
S$8443
  Bottom 0: 175.54,137.12 175.19,137.41
S$8444
  Bottom 0: 175.19,137.41 174.8,137.62
S$8445
  Bottom 0: 174.8,137.62 174.37,137.75
S$8446
  Bottom 0: 174.37,137.75 173.92,137.79
S$8447
  Bottom 0: 173.92,137.79 173.48,137.75
S$8448
  Bottom 0: 173.48,137.75 173.05,137.62
S$8449
  Bottom 0: 173.05,137.62 172.65,137.41
S$8450
  Bottom 0: 172.65,137.41 172.31,137.12
S$8451
  Bottom 0: 172.31,137.12 172.02,136.78
S$8452
  Bottom 0: 172.02,136.78 171.81,136.38
S$8453
  Bottom 0: 171.81,136.38 171.68,135.96
S$8454
  Bottom 0: 171.68,135.96 171.64,135.51
S$8455
  Bottom 0: 171.64,135.51 171.68,135.06
S$8456
  Bottom 0: 171.68,135.06 171.81,134.63
S$8457
  Bottom 0: 171.81,134.63 172.02,134.24
S$8458
  Bottom 0: 172.02,134.24 172.31,133.89
S$8459
  Bottom 0: 172.31,133.89 172.65,133.61
S$8460
  Bottom 0: 172.65,133.61 173.05,133.4
S$8461
  Bottom 0: 173.05,133.4 173.48,133.27
S$8462
  Bottom 0: 173.48,133.27 173.92,133.22
S$8463
  Bottom 0: 164.5,138.54 164.79,138.61
S$8464
  Bottom 0: 164.79,138.61 165.05,138.76
S$8465
  Bottom 0: 165.05,138.76 165.26,138.98
S$8466
  Bottom 0: 165.26,138.98 165.39,139.25
S$8467
  Bottom 0: 165.39,139.25 165.44,139.55
S$8468
  Bottom 0: 165.44,139.55 165.39,139.85
S$8469
  Bottom 0: 165.39,139.85 165.26,140.13
S$8470
  Bottom 0: 165.26,140.13 165.05,140.34
S$8471
  Bottom 0: 165.05,140.34 164.79,140.5
S$8472
  Bottom 0: 164.79,140.5 164.5,140.56
S$8473
  Bottom 0: 164.5,140.56 164.19,140.54
S$8474
  Bottom 0: 164.19,140.54 163.91,140.43
S$8475
  Bottom 0: 163.91,140.43 163.67,140.24
S$8476
  Bottom 0: 163.67,140.24 163.5,140
S$8477
  Bottom 0: 163.5,140 163.41,139.71
S$8478
  Bottom 0: 163.41,139.71 163.41,139.4
S$8479
  Bottom 0: 163.41,139.4 163.5,139.11
S$8480
  Bottom 0: 163.5,139.11 163.67,138.86
S$8481
  Bottom 0: 163.67,138.86 163.91,138.67
S$8482
  Bottom 0: 163.91,138.67 164.19,138.56
S$8483
  Bottom 0: 164.19,138.56 164.5,138.54
S$8484
  Bottom 0: 171.76,139.45 173.54,139.45
S$8485
  Bottom 0: 173.54,139.45 173.62,139.46
S$8486
  Bottom 0: 173.62,139.46 173.69,139.5
S$8487
  Bottom 0: 173.69,139.5 173.75,139.55
S$8488
  Bottom 0: 173.75,139.55 173.79,139.62
S$8489
  Bottom 0: 173.79,139.62 173.8,139.7
S$8490
  Bottom 0: 173.8,139.7 173.8,141.48
S$8491
  Bottom 0: 173.8,141.48 173.79,141.55
S$8492
  Bottom 0: 173.79,141.55 173.75,141.62
S$8493
  Bottom 0: 173.75,141.62 173.69,141.68
S$8494
  Bottom 0: 173.69,141.68 173.62,141.72
S$8495
  Bottom 0: 173.62,141.72 173.54,141.73
S$8496
  Bottom 0: 173.54,141.73 173.1,141.73
S$8497
  Bottom 0: 173.1,141.73 173.1,141.86
S$8498
  Bottom 0: 173.1,141.86 173.03,142.08
S$8499
  Bottom 0: 173.03,142.08 172.87,142.24
S$8500
  Bottom 0: 172.87,142.24 172.65,142.3
S$8501
  Bottom 0: 172.65,142.3 172.3,142.3
S$8502
  Bottom 0: 172.3,142.3 171.22,143.38
S$8503
  Bottom 0: 171.22,143.38 171.28,143.52
S$8504
  Bottom 0: 171.28,143.52 171.33,143.84
S$8505
  Bottom 0: 171.33,143.84 171.28,144.16
S$8506
  Bottom 0: 171.28,144.16 171.15,144.46
S$8507
  Bottom 0: 171.15,144.46 170.95,144.71
S$8508
  Bottom 0: 170.95,144.71 170.68,144.9
S$8509
  Bottom 0: 170.68,144.9 170.38,145.01
S$8510
  Bottom 0: 170.38,145.01 170.05,145.03
S$8511
  Bottom 0: 170.05,145.03 169.73,144.96
S$8512
  Bottom 0: 169.73,144.96 169.44,144.82
S$8513
  Bottom 0: 169.44,144.82 169.21,144.59
S$8514
  Bottom 0: 169.21,144.59 169.04,144.32
S$8515
  Bottom 0: 169.04,144.32 168.95,144
S$8516
  Bottom 0: 168.95,144 168.95,143.68
S$8517
  Bottom 0: 168.95,143.68 169.04,143.36
S$8518
  Bottom 0: 169.04,143.36 169.21,143.09
S$8519
  Bottom 0: 169.21,143.09 169.44,142.87
S$8520
  Bottom 0: 169.44,142.87 169.73,142.72
S$8521
  Bottom 0: 169.73,142.72 170.05,142.65
S$8522
  Bottom 0: 170.05,142.65 170.38,142.67
S$8523
  Bottom 0: 170.38,142.67 170.6,142.75
S$8524
  Bottom 0: 170.6,142.75 171.65,141.7
S$8525
  Bottom 0: 171.65,141.7 171.62,141.68
S$8526
  Bottom 0: 171.62,141.68 171.56,141.62
S$8527
  Bottom 0: 171.56,141.62 171.52,141.55
S$8528
  Bottom 0: 171.52,141.55 171.51,141.48
S$8529
  Bottom 0: 171.51,141.48 171.51,139.7
S$8530
  Bottom 0: 171.51,139.7 171.52,139.62
S$8531
  Bottom 0: 171.52,139.62 171.56,139.55
S$8532
  Bottom 0: 171.56,139.55 171.62,139.5
S$8533
  Bottom 0: 171.62,139.5 171.69,139.46
S$8534
  Bottom 0: 171.69,139.46 171.76,139.45
S$8535
  Bottom 0: 175.03,139.46 175.36,139.46
S$8536
  Bottom 0: 175.36,139.46 175.66,139.55
S$8537
  Bottom 0: 175.66,139.55 175.94,139.72
S$8538
  Bottom 0: 175.94,139.72 176.15,139.97
S$8539
  Bottom 0: 176.15,139.97 176.29,140.27
S$8540
  Bottom 0: 176.29,140.27 176.34,140.59
S$8541
  Bottom 0: 176.34,140.59 176.29,140.91
S$8542
  Bottom 0: 176.29,140.91 176.15,141.21
S$8543
  Bottom 0: 176.15,141.21 175.94,141.45
S$8544
  Bottom 0: 175.94,141.45 175.66,141.63
S$8545
  Bottom 0: 175.66,141.63 175.36,141.72
S$8546
  Bottom 0: 175.36,141.72 175.03,141.72
S$8547
  Bottom 0: 175.03,141.72 174.72,141.63
S$8548
  Bottom 0: 174.72,141.63 174.45,141.45
S$8549
  Bottom 0: 174.45,141.45 174.23,141.21
S$8550
  Bottom 0: 174.23,141.21 174.1,140.91
S$8551
  Bottom 0: 174.1,140.91 174.05,140.59
S$8552
  Bottom 0: 174.05,140.59 174.1,140.27
S$8553
  Bottom 0: 174.1,140.27 174.23,139.97
S$8554
  Bottom 0: 174.23,139.97 174.45,139.72
S$8555
  Bottom 0: 174.45,139.72 174.72,139.55
S$8556
  Bottom 0: 174.72,139.55 175.03,139.46
S$8557
  Bottom 0: 275.51,101.93 271.65,105.79
S$8558
  Bottom 0: 271.65,105.79 271.65,114.74
S$8559
  Bottom 0: 271.65,114.74 272.07,114.33
S$8560
  Bottom 0: 272.07,114.33 272.06,114.33
S$8561
  Bottom 0: 272.06,114.33 271.99,114.28
S$8562
  Bottom 0: 271.99,114.28 271.94,114.23
S$8563
  Bottom 0: 271.94,114.23 271.9,114.16
S$8564
  Bottom 0: 271.9,114.16 271.89,114.08
S$8565
  Bottom 0: 271.89,114.08 271.89,111.68
S$8566
  Bottom 0: 271.89,111.68 271.9,111.61
S$8567
  Bottom 0: 271.9,111.61 271.94,111.54
S$8568
  Bottom 0: 271.94,111.54 271.99,111.48
S$8569
  Bottom 0: 271.99,111.48 272.06,111.44
S$8570
  Bottom 0: 272.06,111.44 272.14,111.43
S$8571
  Bottom 0: 272.14,111.43 272.94,111.43
S$8572
  Bottom 0: 272.94,111.43 273.01,111.44
S$8573
  Bottom 0: 273.01,111.44 273.09,111.48
S$8574
  Bottom 0: 273.09,111.48 273.14,111.54
S$8575
  Bottom 0: 273.14,111.54 273.18,111.59
S$8576
  Bottom 0: 273.18,111.59 273.2,111.54
S$8577
  Bottom 0: 273.2,111.54 273.26,111.48
S$8578
  Bottom 0: 273.26,111.48 273.33,111.44
S$8579
  Bottom 0: 273.33,111.44 273.41,111.43
S$8580
  Bottom 0: 273.41,111.43 273.61,111.43
S$8581
  Bottom 0: 273.61,111.43 273.61,112.28
S$8582
  Bottom 0: 273.61,112.28 273.19,112.28
S$8583
  Bottom 0: 273.19,112.28 273.19,113.48
S$8584
  Bottom 0: 273.19,113.48 273.61,113.48
S$8585
  Bottom 0: 273.61,113.48 273.61,114.34
S$8586
  Bottom 0: 273.61,114.34 273.41,114.34
S$8587
  Bottom 0: 273.41,114.34 273.33,114.33
S$8588
  Bottom 0: 273.33,114.33 273.26,114.28
S$8589
  Bottom 0: 273.26,114.28 273.2,114.23
S$8590
  Bottom 0: 273.2,114.23 273.18,114.17
S$8591
  Bottom 0: 273.18,114.17 273.14,114.23
S$8592
  Bottom 0: 273.14,114.23 273.09,114.28
S$8593
  Bottom 0: 273.09,114.28 273.01,114.33
S$8594
  Bottom 0: 273.01,114.33 272.98,114.33
S$8595
  Bottom 0: 272.98,114.33 272.98,114.48
S$8596
  Bottom 0: 272.98,114.48 272.97,114.53
S$8597
  Bottom 0: 272.97,114.53 272.97,114.59
S$8598
  Bottom 0: 272.97,114.59 272.94,114.64
S$8599
  Bottom 0: 272.94,114.64 272.92,114.7
S$8600
  Bottom 0: 272.92,114.7 272.88,114.74
S$8601
  Bottom 0: 272.88,114.74 272.85,114.79
S$8602
  Bottom 0: 272.85,114.79 272.21,115.43
S$8603
  Bottom 0: 272.21,115.43 272.21,115.72
S$8604
  Bottom 0: 272.21,115.72 272.24,115.7
S$8605
  Bottom 0: 272.24,115.7 272.29,115.66
S$8606
  Bottom 0: 272.29,115.66 272.36,115.65
S$8607
  Bottom 0: 272.36,115.65 272.42,115.62
S$8608
  Bottom 0: 272.42,115.62 272.48,115.62
S$8609
  Bottom 0: 272.48,115.62 272.54,115.61
S$8610
  Bottom 0: 272.54,115.61 276.12,115.61
S$8611
  Bottom 0: 276.12,115.61 276.69,115.03
S$8612
  Bottom 0: 276.69,115.03 276.69,114.34
S$8613
  Bottom 0: 276.69,114.34 276.55,114.34
S$8614
  Bottom 0: 276.55,114.34 276.55,113.48
S$8615
  Bottom 0: 276.55,113.48 276.69,113.48
S$8616
  Bottom 0: 276.69,113.48 276.69,112.28
S$8617
  Bottom 0: 276.69,112.28 276.55,112.28
S$8618
  Bottom 0: 276.55,112.28 276.55,111.43
S$8619
  Bottom 0: 276.55,111.43 276.69,111.43
S$8620
  Bottom 0: 276.69,111.43 276.69,111.02
S$8621
  Bottom 0: 276.69,111.02 276.69,110.93
S$8622
  Bottom 0: 276.69,110.93 276.72,110.84
S$8623
  Bottom 0: 276.72,110.84 276.75,110.76
S$8624
  Bottom 0: 276.75,110.76 276.8,110.68
S$8625
  Bottom 0: 276.8,110.68 276.86,110.62
S$8626
  Bottom 0: 276.86,110.62 281.4,106.07
S$8627
  Bottom 0: 281.4,106.07 281.36,105.9
S$8628
  Bottom 0: 281.36,105.9 281.36,105.57
S$8629
  Bottom 0: 281.36,105.57 281.44,105.26
S$8630
  Bottom 0: 281.44,105.26 281.62,104.98
S$8631
  Bottom 0: 281.62,104.98 281.85,104.76
S$8632
  Bottom 0: 281.85,104.76 282.14,104.61
S$8633
  Bottom 0: 282.14,104.61 282.46,104.55
S$8634
  Bottom 0: 282.46,104.55 282.78,104.57
S$8635
  Bottom 0: 282.78,104.57 283.09,104.67
S$8636
  Bottom 0: 283.09,104.67 283.35,104.86
S$8637
  Bottom 0: 283.35,104.86 283.56,105.11
S$8638
  Bottom 0: 283.56,105.11 283.69,105.42
S$8639
  Bottom 0: 283.69,105.42 283.73,105.73
S$8640
  Bottom 0: 283.73,105.73 283.69,106.06
S$8641
  Bottom 0: 283.69,106.06 283.56,106.36
S$8642
  Bottom 0: 283.56,106.36 283.35,106.61
S$8643
  Bottom 0: 283.35,106.61 283.09,106.8
S$8644
  Bottom 0: 283.09,106.8 282.78,106.9
S$8645
  Bottom 0: 282.78,106.9 282.46,106.92
S$8646
  Bottom 0: 282.46,106.92 282.2,106.87
S$8647
  Bottom 0: 282.2,106.87 277.83,111.25
S$8648
  Bottom 0: 277.83,111.25 277.83,115.27
S$8649
  Bottom 0: 277.83,115.27 277.82,115.36
S$8650
  Bottom 0: 277.82,115.36 277.81,115.44
S$8651
  Bottom 0: 277.81,115.44 277.77,115.52
S$8652
  Bottom 0: 277.77,115.52 277.72,115.6
S$8653
  Bottom 0: 277.72,115.6 277.66,115.67
S$8654
  Bottom 0: 277.66,115.67 276.92,116.41
S$8655
  Bottom 0: 276.92,116.41 276.92,116.5
S$8656
  Bottom 0: 276.92,116.5 276.95,116.53
S$8657
  Bottom 0: 276.95,116.53 276.99,116.61
S$8658
  Bottom 0: 276.99,116.61 277,116.68
S$8659
  Bottom 0: 277,116.68 277,118.88
S$8660
  Bottom 0: 277,118.88 280.12,115.75
S$8661
  Bottom 0: 280.12,115.75 280.12,115.74
S$8662
  Bottom 0: 280.12,115.74 280.14,115.74
S$8663
  Bottom 0: 280.14,115.74 280.66,115.22
S$8664
  Bottom 0: 280.66,115.22 280.66,113.76
S$8665
  Bottom 0: 280.66,113.76 280.41,113.64
S$8666
  Bottom 0: 280.41,113.64 280.18,113.41
S$8667
  Bottom 0: 280.18,113.41 280,113.14
S$8668
  Bottom 0: 280,113.14 279.92,112.82
S$8669
  Bottom 0: 279.92,112.82 279.92,112.5
S$8670
  Bottom 0: 279.92,112.5 280,112.18
S$8671
  Bottom 0: 280,112.18 280.18,111.91
S$8672
  Bottom 0: 280.18,111.91 280.41,111.68
S$8673
  Bottom 0: 280.41,111.68 280.7,111.54
S$8674
  Bottom 0: 280.7,111.54 281.02,111.47
S$8675
  Bottom 0: 281.02,111.47 281.35,111.49
S$8676
  Bottom 0: 281.35,111.49 281.65,111.6
S$8677
  Bottom 0: 281.65,111.6 281.92,111.78
S$8678
  Bottom 0: 281.92,111.78 282.12,112.04
S$8679
  Bottom 0: 282.12,112.04 282.25,112.34
S$8680
  Bottom 0: 282.25,112.34 282.3,112.66
S$8681
  Bottom 0: 282.3,112.66 282.25,112.98
S$8682
  Bottom 0: 282.25,112.98 282.12,113.28
S$8683
  Bottom 0: 282.12,113.28 281.92,113.53
S$8684
  Bottom 0: 281.92,113.53 281.65,113.72
S$8685
  Bottom 0: 281.65,113.72 281.54,113.76
S$8686
  Bottom 0: 281.54,113.76 281.54,115.4
S$8687
  Bottom 0: 281.54,115.4 281.54,115.47
S$8688
  Bottom 0: 281.54,115.47 281.52,115.54
S$8689
  Bottom 0: 281.52,115.54 281.49,115.61
S$8690
  Bottom 0: 281.49,115.61 281.45,115.66
S$8691
  Bottom 0: 281.45,115.66 281.41,115.72
S$8692
  Bottom 0: 281.41,115.72 281.07,116.06
S$8693
  Bottom 0: 281.07,116.06 284.21,119.19
S$8694
  Bottom 0: 284.21,119.19 284.27,119.16
S$8695
  Bottom 0: 284.27,119.16 284.59,119.1
S$8696
  Bottom 0: 284.59,119.1 284.91,119.12
S$8697
  Bottom 0: 284.91,119.12 285.22,119.22
S$8698
  Bottom 0: 285.22,119.22 285.48,119.41
S$8699
  Bottom 0: 285.48,119.41 285.69,119.66
S$8700
  Bottom 0: 285.69,119.66 285.82,119.96
S$8701
  Bottom 0: 285.82,119.96 285.86,120.28
S$8702
  Bottom 0: 285.86,120.28 285.82,120.6
S$8703
  Bottom 0: 285.82,120.6 285.69,120.9
S$8704
  Bottom 0: 285.69,120.9 285.48,121.16
S$8705
  Bottom 0: 285.48,121.16 285.22,121.35
S$8706
  Bottom 0: 285.22,121.35 284.91,121.45
S$8707
  Bottom 0: 284.91,121.45 284.59,121.47
S$8708
  Bottom 0: 284.59,121.47 284.27,121.41
S$8709
  Bottom 0: 284.27,121.41 283.98,121.26
S$8710
  Bottom 0: 283.98,121.26 283.74,121.04
S$8711
  Bottom 0: 283.74,121.04 283.57,120.76
S$8712
  Bottom 0: 283.57,120.76 283.48,120.45
S$8713
  Bottom 0: 283.48,120.45 283.48,120.12
S$8714
  Bottom 0: 283.48,120.12 283.57,119.82
S$8715
  Bottom 0: 283.57,119.82 280.44,116.69
S$8716
  Bottom 0: 280.44,116.69 277.37,119.76
S$8717
  Bottom 0: 277.37,119.76 277.31,119.81
S$8718
  Bottom 0: 277.31,119.81 277.26,119.84
S$8719
  Bottom 0: 277.26,119.84 277.19,119.87
S$8720
  Bottom 0: 277.19,119.87 277.12,119.89
S$8721
  Bottom 0: 277.12,119.89 277.05,119.89
S$8722
  Bottom 0: 277.05,119.89 271.88,119.89
S$8723
  Bottom 0: 271.88,119.89 271.81,119.89
S$8724
  Bottom 0: 271.81,119.89 271.74,119.87
S$8725
  Bottom 0: 271.74,119.87 271.68,119.85
S$8726
  Bottom 0: 271.68,119.85 271.65,119.83
S$8727
  Bottom 0: 271.65,119.83 271.65,129.3
S$8728
  Bottom 0: 271.65,129.3 283.49,141.14
S$8729
  Bottom 0: 283.49,141.14 283.69,141.13
S$8730
  Bottom 0: 283.69,141.13 283.93,141.19
S$8731
  Bottom 0: 283.93,141.19 284.14,141.35
S$8732
  Bottom 0: 284.14,141.35 284.27,141.56
S$8733
  Bottom 0: 284.27,141.56 284.31,141.81
S$8734
  Bottom 0: 284.31,141.81 284.27,142.06
S$8735
  Bottom 0: 284.27,142.06 284.14,142.27
S$8736
  Bottom 0: 284.14,142.27 283.98,142.39
S$8737
  Bottom 0: 283.98,142.39 283.98,146.75
S$8738
  Bottom 0: 283.98,146.75 283.97,146.82
S$8739
  Bottom 0: 283.97,146.82 283.96,146.89
S$8740
  Bottom 0: 283.96,146.89 283.93,146.95
S$8741
  Bottom 0: 283.93,146.95 283.89,147.01
S$8742
  Bottom 0: 283.89,147.01 283.85,147.07
S$8743
  Bottom 0: 283.85,147.07 273.74,157.18
S$8744
  Bottom 0: 273.74,157.18 275.31,157.18
S$8745
  Bottom 0: 275.31,157.18 286.22,146.26
S$8746
  Bottom 0: 286.22,146.26 286.22,146.1
S$8747
  Bottom 0: 286.22,146.1 286.31,145.86
S$8748
  Bottom 0: 286.31,145.86 286.49,145.67
S$8749
  Bottom 0: 286.49,145.67 286.71,145.56
S$8750
  Bottom 0: 286.71,145.56 286.96,145.54
S$8751
  Bottom 0: 286.96,145.54 287.2,145.61
S$8752
  Bottom 0: 287.2,145.61 287.41,145.76
S$8753
  Bottom 0: 287.41,145.76 287.54,145.97
S$8754
  Bottom 0: 287.54,145.97 287.58,146.22
S$8755
  Bottom 0: 287.58,146.22 287.54,146.47
S$8756
  Bottom 0: 287.54,146.47 287.41,146.69
S$8757
  Bottom 0: 287.41,146.69 287.2,146.84
S$8758
  Bottom 0: 287.2,146.84 286.96,146.9
S$8759
  Bottom 0: 286.96,146.9 286.85,146.89
S$8760
  Bottom 0: 286.85,146.89 275.82,157.93
S$8761
  Bottom 0: 275.82,157.93 276.43,157.93
S$8762
  Bottom 0: 276.43,157.93 276.44,157.89
S$8763
  Bottom 0: 276.44,157.89 276.62,157.62
S$8764
  Bottom 0: 276.62,157.62 276.85,157.39
S$8765
  Bottom 0: 276.85,157.39 277.14,157.25
S$8766
  Bottom 0: 277.14,157.25 277.46,157.18
S$8767
  Bottom 0: 277.46,157.18 277.79,157.2
S$8768
  Bottom 0: 277.79,157.2 278.09,157.31
S$8769
  Bottom 0: 278.09,157.31 278.35,157.49
S$8770
  Bottom 0: 278.35,157.49 278.56,157.75
S$8771
  Bottom 0: 278.56,157.75 278.69,158.05
S$8772
  Bottom 0: 278.69,158.05 278.74,158.37
S$8773
  Bottom 0: 278.74,158.37 278.69,158.69
S$8774
  Bottom 0: 278.69,158.69 278.56,158.99
S$8775
  Bottom 0: 278.56,158.99 278.35,159.24
S$8776
  Bottom 0: 278.35,159.24 278.09,159.43
S$8777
